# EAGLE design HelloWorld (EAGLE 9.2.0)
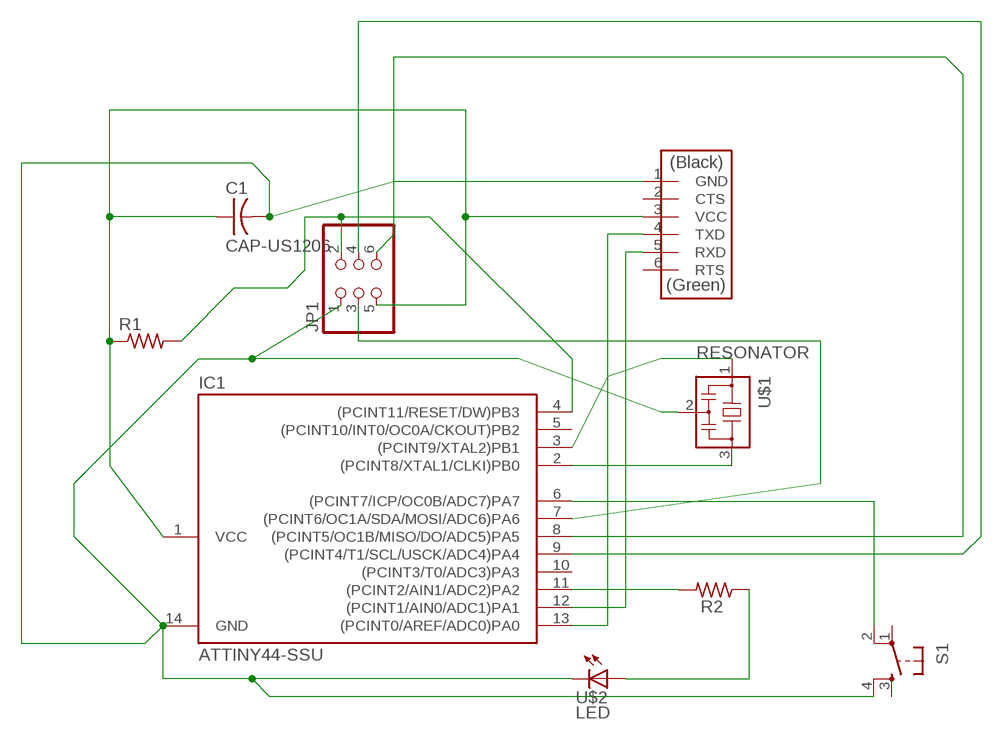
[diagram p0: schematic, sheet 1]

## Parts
C1  CAP-US1206  [C1206]
IC1  ATTINY44-SSU  [SOIC14]
JP1  PINHD-2X3-SMD  [2X03SMD]
R1  RES-US1206  [R1206]
R2  RES-US1206  [R1206]
S1  6MM_SWITCH6MM_SWITCH  [6MM_SWITCH]
U$1  RESONATOR  [EFOBM]
U$2  LED  [LED1206]
U$3  FTDI-SMD-HEADER  [1X06SMD]

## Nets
N$1: IC1.13((PCINT0/AREF/ADC0)PA0) U$3.4(TXD)
N$2: IC1.2((PCINT8/XTAL1/CLKI)PB0) U$1.3
N$3: IC1.4((PCINT11/RESET/DW)PB3) JP1.2 R1.2
N$4: IC1.3((PCINT9/XTAL2)PB1) U$1.1
N$5: C1.2 IC1.14(GND) JP1.1 S1.4(S1) U$1.2 U$2.2(C) U$3.1(GND)
N$6: C1.1 IC1.1(VCC) JP1.5 R1.1 U$3.3(VCC)
N$7: IC1.12((PCINT1/AIN0/ADC1)PA1) U$3.5(RXD)
N$8: IC1.7((PCINT6/OC1A/SDA/MOSI/ADC6)PA6) JP1.3
N$9: IC1.9((PCINT4/T1/SCL/USCK/ADC4)PA4) JP1.4
N$10: IC1.8((PCINT5/OC1B/MISO/DO/ADC5)PA5) JP1.6
N$11: IC1.11((PCINT2/AIN1/ADC2)PA2) R2.2
N$12: R2.1 U$2.1(A)
N$13: IC1.6((PCINT7/ICP/OC0B/ADC7)PA7) S1.2(P1)
Unconnected: IC1.5((PCINT10/INT0/OC0A/CKOUT)PB2) IC1.10((PCINT3/T0/ADC3)PA3) S1.1(P) S1.3(S) U$3.2(CTS) U$3.6(RTS)

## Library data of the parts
C1 = fab:CAP-US
IC1 = fab:ATTINY44
JP1 = fab:PINHD-2X3-SMD: PIN HEADER
R1 R2 = fab:RES-US: Resistor (US Symbol)
S1 = fab:6MM_SWITCH: OMRON SWITCH
U$1 = fab:RESONATOR
U$2 = fab:LED: LED
U$3 = fab:FTDI-SMD-HEADER

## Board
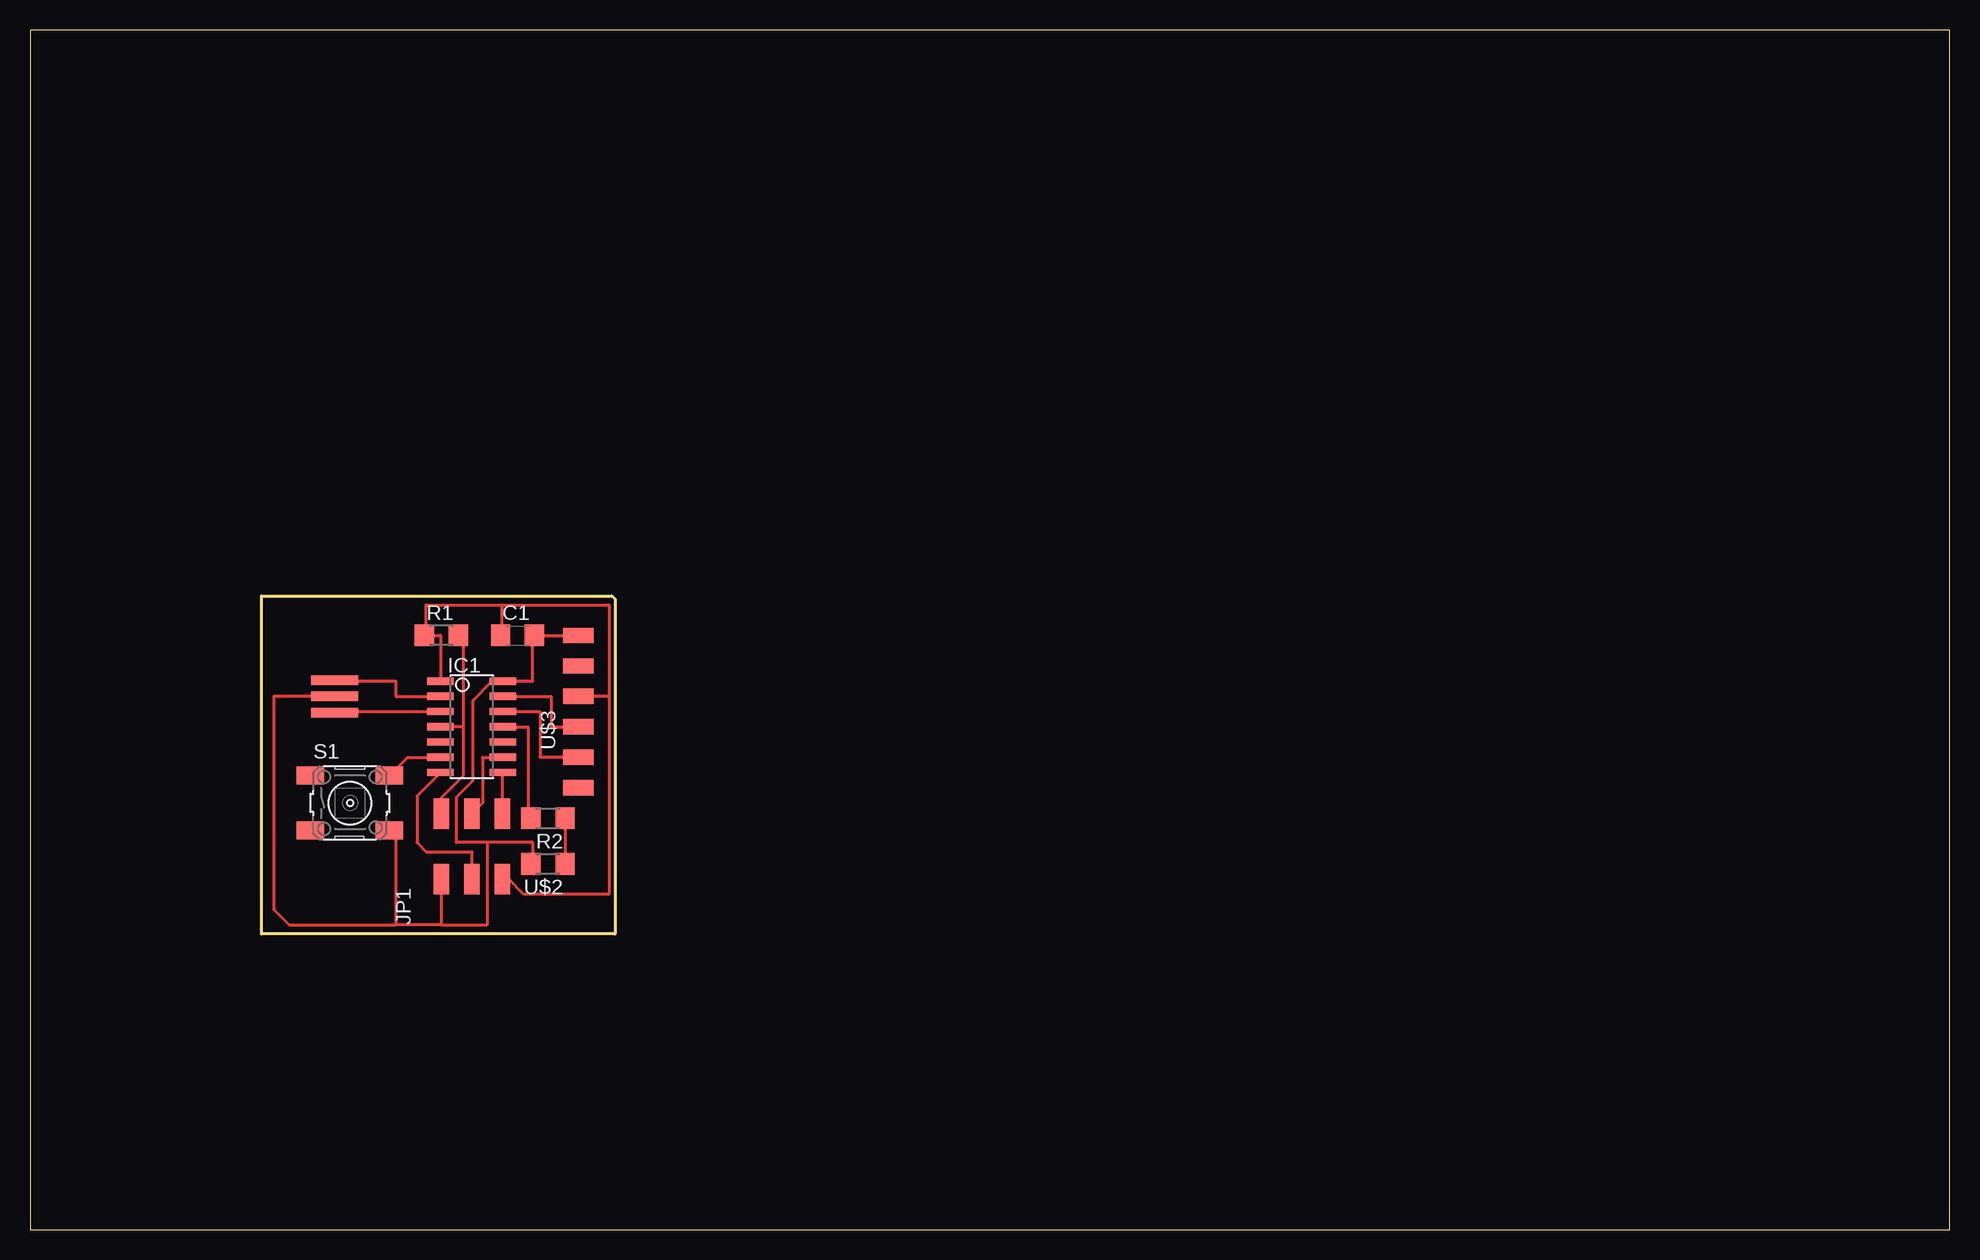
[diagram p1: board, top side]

Size 160 x 100 mm. Coordinates in mm from the lower left corner, seen from the top.
Outline: 0,0 160,0 160,100 0,100 0,0
Copper layers (1*16): Top 0.035mm / dielectric 1.5mm / Bottom 0.035mm
Design rules "fabcity-designrules": minimum track width 10mil, minimum drill 32mil, track to track 16mil, track to pad 16mil, pad to pad 16mil, via to via 16mil, smd to smd 6mil, copper to edge 16mil, drill to drill 16mil, minimum pad ring 10mil, minimum via ring 8mil, stop-mask expansion 4mil, vias tented up to drill 0mil, thermal gap 16mil
Milling: area 19.3,24.6 to 48.8,52.8

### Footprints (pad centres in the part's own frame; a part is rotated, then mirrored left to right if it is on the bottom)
C1206 = smd 1.6 x 1.8: 1 -1.4,0; 2 1.4,0
SOIC14 = smd 0.61 x 2.21: 1 -3.81,-2.603; 2 -2.54,-2.603; 3 -1.27,-2.603; 4 0,-2.603; 5 1.27,-2.603; 6 2.54,-2.603; 7 3.81,-2.603; 8 3.81,2.603; 9 2.54,2.603; 10 1.27,2.603; 11 0,2.603; 12 -1.27,2.603; 13 -2.54,2.603; 14 -3.81,2.603
2X03SMD = smd 2.54 x 1.27: 1 -2.54,2.54; 2 2.92,2.54; 3 -2.54,0; 4 2.92,0; 5 -2.54,-2.54; 6 2.92,-2.54
R1206 = smd 1.6 x 1.803: 1 -1.422,0; 2 1.422,0
6MM_SWITCH = smd 2.286 x 1.524: 1 -3.302,2.286; 2 3.302,2.286; 3 -3.302,-2.286; 4 3.302,-2.286
EFOBM = smd 0.8 x 3.9: 1 -1.35,0; 2 0,0; 3 1.35,0
LED1206 = smd 1.6 x 1.803: 1 -1.422,0; 2 1.422,0
1X06SMD = smd 2.54 x 1.27: 1 0,6.35; 2 0,3.81; 3 0,1.27; 4 0,-1.27; 5 0,-3.81; 6 0,-6.35

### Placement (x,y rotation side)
C1  40.64,49.53 0 top
IC1  36.83,41.91 270 top
JP1  36.83,31.75 90 top
R1  34.29,49.53 0 top
R2  43.18,34.29 180 top
S1  26.67,35.56 0 top
U$1  25.4,44.45 90 top
U$2  43.18,30.48 180 top
U$3  45.72,43.18 0 top

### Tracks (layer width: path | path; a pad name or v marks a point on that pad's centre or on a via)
N$1
  Top 0.254: IC1.13 43.43,44.45 43.43,41.91 U$3.4
N$2
  Top 0.254: U$1.3 25.48,45.72 30.48,45.72 30.48,44.45 IC1.2
N$3
  Top 0.254: 36.12,41.91 36.12,37.83 34.29,36 JP1.2 | 36.12,41.91 IC1.4 | R1.2 36.12,49.12 36.12,41.91
N$4
  Top 0.254: U$1.1 25.48,43.18 IC1.3
N$5
  Top 0.254: U$1.2 20.32,44.45 20.32,26.67 21.59,25.4 30.48,25.4 | 34.29,25.4 30.48,25.4 | S1.4 30.48,32.77 30.48,25.4 | JP1.1 34.29,25.4 | 34.29,25.4 38.1,25.4 38.1,32.26 | 38.1,32.26 41.91,32.26 41.91,30.63 U$2.2 | U$3.1 C1.2 41.91,49.4 41.91,45.72 IC1.14 38.54,45.72 36.93,44.11 36.93,37.43 35.53,36.03 35.53,32.26 38.1,32.26
N$6
  Top 0.254: 39.37,52.07 33.02,52.07 33.02,49.68 R1.1 34.23,49.53 IC1.1 | C1.1 39.37,49.66 39.37,52.07 | 39.37,52.07 48.26,52.07 48.26,44.45 | 48.26,44.45 U$3.3 | 48.26,44.45 48.26,27.94 41.15,27.94 39.88,29.21 JP1.5
N$7
  Top 0.254: IC1.12 42.52,43.18 42.52,39.37 U$3.5
N$8
  Top 0.254: IC1.7 32.26,36.13 32.26,32.26 33.02,31.5 36.83,31.5 JP1.3
N$9
  Top 0.254: JP1.4 37.72,35.56 37.72,39.37 IC1.9
N$10
  Top 0.254: IC1.8 39.37,38.04 JP1.6
N$11
  Top 0.254: IC1.11 41.5,41.91 41.5,34.54 R2.2
N$12
  Top 0.254: R2.1 U$2.1
N$13
  Top 0.254: S1.2 31.5,39.37 IC1.6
